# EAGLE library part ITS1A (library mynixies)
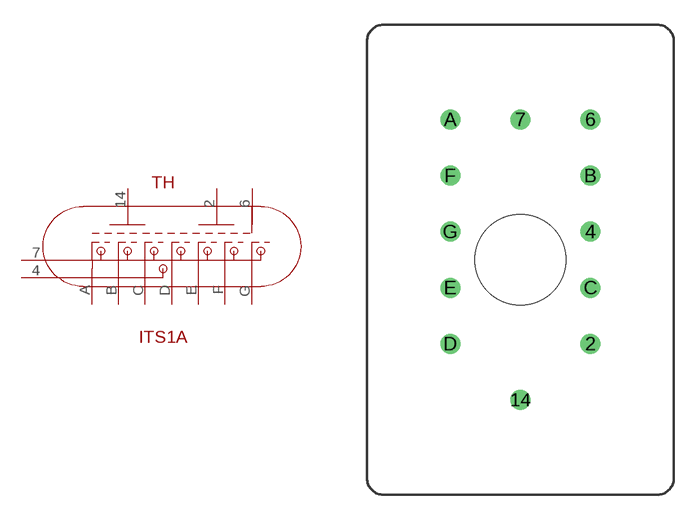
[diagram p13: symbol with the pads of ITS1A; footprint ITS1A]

Designator prefix TH

## ITS1A  [ITS1A]
2  2  pwr
4  4  pwr
6  6  pas
7  7  pwr
14  14  pwr
A  A  pas
B  B  pas
C  C  pas
D  D  pas
E  E  pas
F  F  pas
G  G  pas

## Footprint ITS1A (pad centres in mm)
drill 0.7: 2 4.25,-5.1; 4 4.25,1.7; 6 4.25,8.5; 7 0,8.5; 14 0,-8.5; A -4.25,8.5; B 4.25,5.1; C 4.25,-1.7; D -4.25,-5.1; E -4.25,-1.7; F -4.25,5.1; G -4.25,1.7
hole 5.5 at 0,0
